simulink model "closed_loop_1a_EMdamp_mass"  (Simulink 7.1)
settings: Solver=FixedStepDiscrete  StartTime=0.0  StopTime=Tend  FixedStep=Ts  MaxStep=Ts  MinStep=Ts/10  RelTol=1e-4
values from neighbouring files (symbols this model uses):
  Kt = 0.06    [lame_dat.m]
  Lt = 0.001    [lame_dat.m]
  Ts = 100e-6    (= 0.0001)    [lame_main.m]
libraries: cstblocks x2, powerlib_extras x1

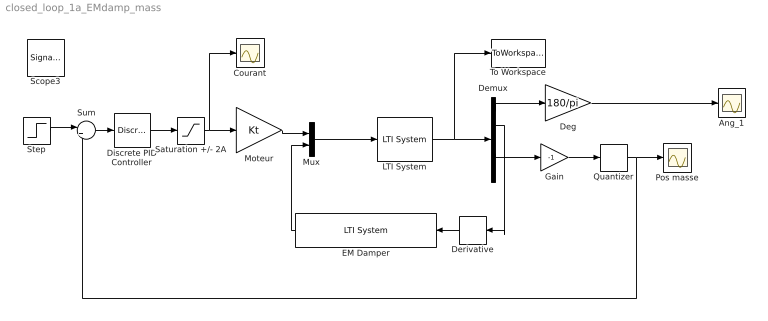
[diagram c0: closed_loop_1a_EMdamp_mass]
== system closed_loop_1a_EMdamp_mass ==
  Ang_1 : Scope
  Courant : Scope
  Deg : Gain  Gain=180/pi  ParameterDataType=fixdt(1, 16)  ParameterScaling=2^0  OutDataType=fixdt(1, 16)  OutScaling=2^0
  Demux : Demux  Outputs=5
  Derivative : Derivative  Orientation=left
  Discrete PID Controller : powerlib_extras/Discrete  Control Blocks/Discrete PID Controller  DialogController=POWERSYS.PowerSysDialog  SystemSampleTime=-1  Kp=1000  Ki=20000  Kd=.3  TcD=Ts  Par_Limits="[1    -1]"  Init=0  Ts=Ts
  EM Damper : cstblocks/LTI System  Orientation=left  SystemSampleTime=-1  sys="c2d(tf(-Kt^2,[Lt  1]),Ts)"  IC=[]
  Gain : Gain  Gain=-1  ParameterDataType=sfix(16)  ParameterScaling=2^0  OutDataType=sfix(16)  OutScaling=2^0
  LTI System : cstblocks/LTI System  SystemSampleTime=-1  sys=sysd  IC=[]
  Moteur : Gain  Gain=Kt  ParameterDataType=sfix(16)  ParameterScaling=2^0  OutDataType=sfix(16)  OutScaling=2^0
  Mux : Mux  Inputs=2
  Pos masse : Scope
  Quantizer : Quantizer  QuantizationInterval=10e-6
  Saturation +/- 2A : Saturate  UpperLimit=2  LowerLimit=-2  OutDataType=sfix(16)  OutScaling=2^0
  Step : Step  Time=0  After=0.001  SampleTime=0
  Sum : Sum  Inputs=|+-  OutDataType=sfix(16)  OutScaling=2^0
  To Workspace : ToWorkspace  VariableName=y_sim_out  SampleTime=-1  SaveFormat=Structure With Time
  Scope3 : SignalViewerScope  IOType=viewer  RefreshTime=0.035000
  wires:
  Deg/1 -> Ang_1/1
  LTI System/1 -> Demux/1, To Workspace/1
  Demux/1 -> Deg/1
  Moteur/1 -> Mux/1
  Mux/1 -> LTI System/1
  Demux/2 -> Derivative/1
  Derivative/1 -> EM Damper/1
  Step/1 -> Sum/1
  Sum/1 -> Discrete PID Controller/1
  Discrete PID Controller/1 -> Saturation +/- 2A/1
  Saturation +/- 2A/1 -> Moteur/1, Courant/1
  Demux/4 -> Gain/1
  EM Damper/1 -> Mux/2
  Quantizer/1 -> Pos masse/1, Sum/2
  Gain/1 -> Quantizer/1
